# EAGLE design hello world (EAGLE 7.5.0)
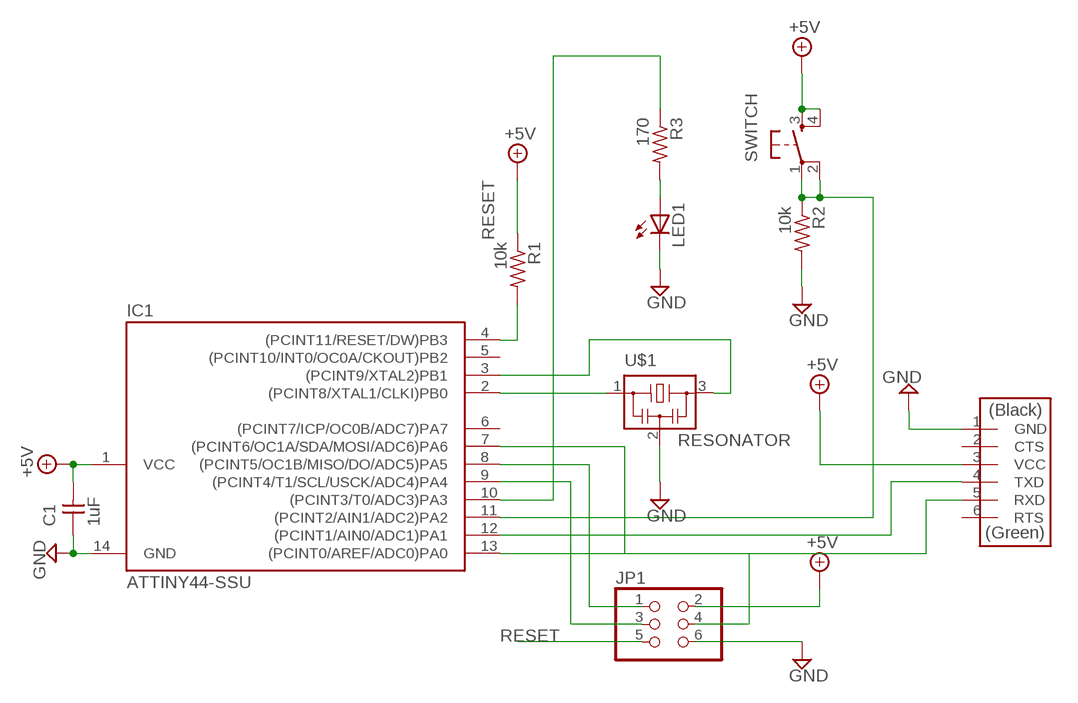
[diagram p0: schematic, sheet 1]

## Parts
C1  1uF  CAP-UNPOLARIZEDFAB  [C1206FAB]
IC1  ATTINY44-SSU  [SOIC14]
JP1  PINHD-2X3-SMD  [2X03SMD]
LED1  LEDP-LCC-2  [P-LCC-2]
R1  10k  RES-US1206FAB  [R1206FAB]
R2  10k  RES-US1206FAB  [R1206FAB]
R3  170  RES-US1206FAB  [R1206FAB]
SWITCH  6MM_SWITCH6MM_SWITCH  [6MM_SWITCH]
U$1  RESONATOR  [EFOBM]
U$2  FTDI-SMD-HEADER  [1X06SMD]

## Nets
+5V: C1.2 IC1.1(VCC) JP1.2 R1.1 SWITCH.3(S) SWITCH.4(S1) U$2.3(VCC)
GND: C1.1 IC1.14(GND) JP1.6 LED1.C R2.2 U$1.2 U$2.1(GND)
N$1: IC1.2((PCINT8/XTAL1/CLKI)PB0) U$1.1
N$2: IC1.3((PCINT9/XTAL2)PB1) U$1.3
N$3: IC1.12((PCINT1/AIN0/ADC1)PA1) U$2.4(TXD)
N$4: IC1.8((PCINT5/OC1B/MISO/DO/ADC5)PA5) JP1.1
N$5: IC1.7((PCINT6/OC1A/SDA/MOSI/ADC6)PA6) JP1.4
N$6: IC1.9((PCINT4/T1/SCL/USCK/ADC4)PA4) JP1.3
N$7: IC1.13((PCINT0/AREF/ADC0)PA0) U$2.5(RXD)
N$8: IC1.11((PCINT2/AIN1/ADC2)PA2) R2.1 SWITCH.1(P) SWITCH.2(P1)
N$10: LED1.A R3.2
N$11: IC1.10((PCINT3/T0/ADC3)PA3) R3.1
RESET: IC1.4((PCINT11/RESET/DW)PB3) JP1.5 R1.2
Unconnected: IC1.5((PCINT10/INT0/OC0A/CKOUT)PB2) IC1.6((PCINT7/ICP/OC0B/ADC7)PA7) U$2.2(CTS) U$2.6(RTS)

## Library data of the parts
C1 = fab:CAP-UNPOLARIZED
IC1 = fab:ATTINY44
JP1 = fab:PINHD-2X3-SMD: PIN HEADER
LED1 = adafruit:LED: LED
R1-R3 = fab:RES-US: Resistor (US Symbol)
SWITCH = fab:6MM_SWITCH: OMRON SWITCH
U$1 = fab:RESONATOR
U$2 = fab:FTDI-SMD-HEADER

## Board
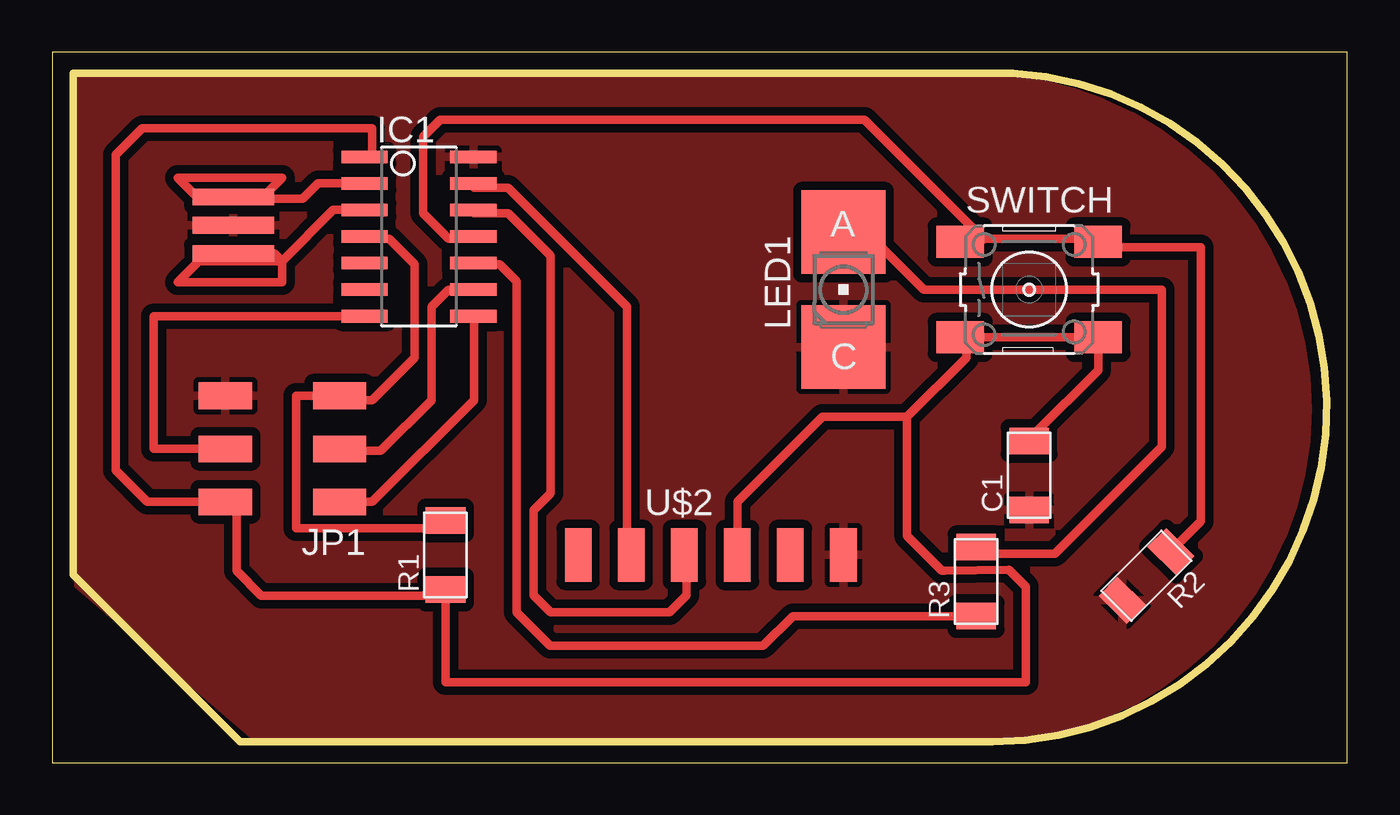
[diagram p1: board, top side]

Size 62 x 34 mm. Coordinates in mm from the lower left corner, seen from the top.
Outline: 0,0 62,0 62,34 0,34 0,0
Copper layers (1*16): Top 0.035mm / dielectric 1.5mm / Bottom 0.035mm
Design rules "default *": minimum track width 16mil, minimum drill 24mil, track to track 16mil, track to pad 16mil, pad to pad 16mil, via to via 16mil, smd to smd 16mil, copper to edge 40mil, drill to drill 8mil, minimum pad ring 10mil, minimum via ring 8mil, stop-mask expansion 4mil, vias tented up to drill 0mil, thermal gap 10mil
Milling: 5 lines

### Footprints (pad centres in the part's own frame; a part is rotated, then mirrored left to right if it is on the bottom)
C1206FAB = smd 1.27 x 1.905: 1 -1.651,0; 2 1.651,0
SOIC14 = smd 0.61 x 2.21: 1 -3.81,-2.603; 2 -2.54,-2.603; 3 -1.27,-2.603; 4 0,-2.603; 5 1.27,-2.603; 6 2.54,-2.603; 7 3.81,-2.603; 8 3.81,2.603; 9 2.54,2.603; 10 1.27,2.603; 11 0,2.603; 12 -1.27,2.603; 13 -2.54,2.603; 14 -3.81,2.603
2X03SMD = smd 2.54 x 1.27: 1 -2.54,2.54; 2 2.92,2.54; 3 -2.54,0; 4 2.92,0; 5 -2.54,-2.54; 6 2.92,-2.54
P-LCC-2 = smd 4 x 4: A 0,2.75; C 0,-2.75
R1206FAB = smd 1.27 x 1.905: 1 -1.651,0; 2 1.651,0
6MM_SWITCH = smd 2.286 x 1.524: 1 -3.302,2.286; 2 3.302,2.286; 3 -3.302,-2.286; 4 3.302,-2.286
EFOBM = smd 0.8 x 3.9: 1 -1.35,0; 2 0,0; 3 1.35,0
1X06SMD = smd 2.54 x 1.27: 1 0,6.35; 2 0,3.81; 3 0,1.27; 4 0,-1.27; 5 0,-3.81; 6 0,-6.35

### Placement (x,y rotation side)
C1  46.77,13.75 90 top
IC1  17.56,25.18 270 top
JP1  11.21,15.02 180 top
LED1  37.88,22.64 0 top
R1  18.83,9.94 90 top
R2  52.39,8.94 225 top
R3  44.23,8.67 90 top
SWITCH  46.77,22.64 0 top
U$1  8.67,25.72 270 top
U$2  31.53,9.94 270 top

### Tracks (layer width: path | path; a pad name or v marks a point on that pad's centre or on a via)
+5V
  Top 0.406: C1.2 47.02,15.73 50.07,18.78 SWITCH.4 | 49.87,20.2 SWITCH.4 | U$2.3 32.8,12.48 36.86,16.54 40.93,16.54 | 40.93,16.54 43.77,19.39 43.77,20.2 SWITCH.3 43.77,20.61 44.03,20.35 SWITCH.4 | IC1.1 15.33,29.14 15.33,30.36 4.3,30.36 3.03,29.09 3.03,13.99 4.54,12.48 JP1.2 8.42,12.48 8.82,12.07 8.82,9.18 10,8 19,8 R1.1 | 40.93,16.54 40.93,10.85 42.6,9.18 42.71,9.18 45.8,9.23 46.62,8.42 46.62,3.86 18.83,3.86 R1.1 | 18.83,6.13 R1.1
GND
  pour Top: 4.86,32.8 44.23,32.8 arc-180 44.23,1.05 9.94,1.05 1.05,8.67 1.05,32.8
N$1
  Top 0.406: IC1.2 12.72,27.72 12,27 10,27 11,28 6,28 7,27 8.6,27 U$1.1 8.67,27
N$2
  Top 0.406: IC1.3 13.45,26.45 11,24 | 11,24 11,23 6,23 7,24 11,24 | 11,24 10.63,24.37 U$1.3
N$3
  Top 0.406: IC1.12 20.2,26.3 21.83,26.3 23.86,24.27 23.86,12.89 23.05,12.07 23.05,8.01 23.86,7.2 29.55,7.2 30.36,8.01 30.36,9.64 U$2.4
N$4
  Top 0.406: JP1.1 15.33,12.48 20.2,17.36 20.2,21.42 IC1.8
N$5
  Top 0.406: JP1.4 4.86,15.02 4.86,21.37 IC1.7
N$6
  Top 0.406: IC1.9 18.98,22.64 18.17,21.83 18.17,17.36 15.73,14.92 14.11,14.92 JP1.3
N$7
  Top 0.406: IC1.13 20.2,27.52 21.83,27.52 27.52,21.83 27.52,10.04 U$2.5
N$8
  Top 0.406: 43.77,24.67 44.18,25.08 44.18,25.48 38.9,30.77 18.58,30.77 17.76,29.95 17.76,26.3 18.98,25.08 19.8,25.08 IC1.11 | 43.77,24.67 44.18,24.67 44.59,25.08 49.87,25.08 SWITCH.2 50.28,24.67 55,24.67 55,11.55 R2.1 | 43.77,24.67 SWITCH.1
N$10
  Top 0.406: 44.59,10.45 R3.2 44.55,10 48,10 53.12,15.12 53.12,22.64 41.74,22.64 39.3,25.08 38.08,25.08 LED1.A
N$11
  Top 0.406: 44.18,6.79 R3.1 35.47,7.02 34.03,5.59 23.84,5.59 22.23,7.2 22.23,23.05 21.42,23.86 20.2,23.86 IC1.10
RESET
  Top 0.406: 13.7,17.76 JP1.5 | IC1.4 15.33,25.08 16.14,25.08 17.36,23.86 17.36,19.39 15.33,17.36 14.11,17.36 JP1.5 | JP1.5 11.67,17.56 11.67,11.26 arc90 11.72,11.21 18.83,11.21 R1.2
